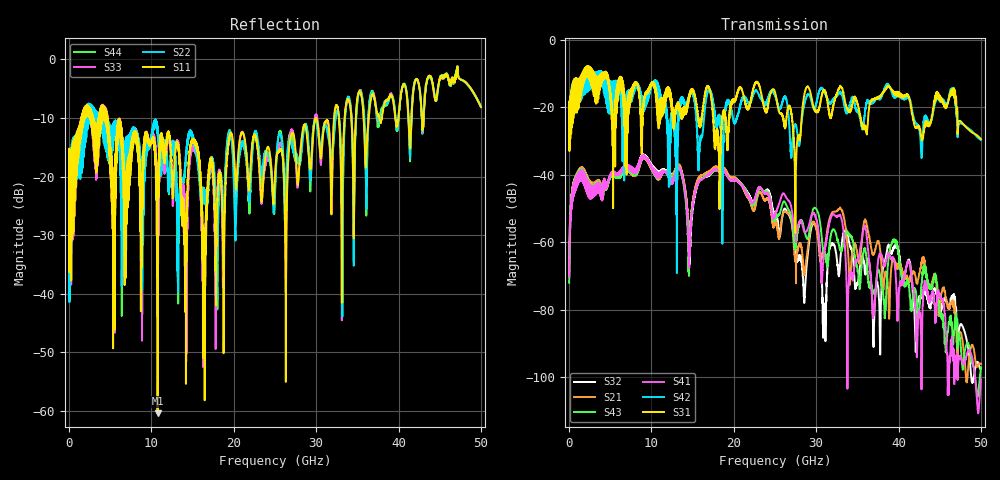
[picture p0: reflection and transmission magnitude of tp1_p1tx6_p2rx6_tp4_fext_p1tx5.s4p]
! 100G CR Analysis
! File: tp1_p1tx6_p2rx6_tp4_fext_p1tx5
! Description: 2m Cu Cable, OSFP, TP1-TP4
! Port Mapping
! Port1 -- P1TX5N
! Port2 -- P2RX6N
! Port3 -- P1TX5P
! Port4 -- P2RX6P
# GHz S MA R 50.00
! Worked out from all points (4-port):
!   5000 points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, 10 MHz to 50 GHz, reference 50 ohm
!   strongest paths, dB at 10 MHz, 12.51 GHz, 25.01 GHz, 37.51 GHz, 50 GHz:
!     S31: -20.6, -20.0, -15.5, -17.2, -29.4
!     S42: -20.5, -20.7, -16.6, -17.4, -29.6
!     S41: -70.0, -42.6, -51.8, -65.8, -100.6
!     S43: -72.0, -42.0, -52.9, -68.5, -97.0
!     S21: -68.5, -40.9, -54.0, -59.8, -96.1
!     S32: -70.3, -40.8, -51.3, -73.1, -97.4
!   lowest |S11| = -60.4 dB at 10.75 GHz (marker M1), VSWR 1.00, Z = 50.1 + j0.0204 ohm
!   |S11| at or under -10 dB: start of sweep to 1.499 GHz; 4.65 GHz to 32.18 GHz (27.53 GHz wide, 149 % of centre); 32.77 GHz to 33.46 GHz (688 MHz wide, 2.08 % of centre)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
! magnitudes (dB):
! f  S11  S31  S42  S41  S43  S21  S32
! 10 MHz  -17.8  -20.6  -20.5  -70.0  -72.0  -68.5  -70.3
! 1.29 GHz  -12.4  -11.5  -11.4  -41.9  -41.2  -40.9  -41.0
! 10.75 GHz  -60.4  -20.5  -12.7  -40.8  -41.0  -41.3  -40.2
! 29.79 GHz  -10.8  -20.7  -20.4  -51.7  -49.7  -54.4  -54.5
! 30.99 GHz  -11.1  -15.0  -15.1  -62.8  -63.3  -61.9  -78.2
! 33.54 GHz  -8.7  -18.6  -20.5  -63.0  -58.2  -55.0  -56.4
! 50 GHz  -8.1  -29.4  -29.6  -100.6  -97.0  -96.1  -97.4
